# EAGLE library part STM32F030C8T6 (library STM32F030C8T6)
32-Bit MCU Cortex-M0 64KB Flash LQFP48 STM32F030C8T6, 32 bit ARM Cortex M0 Microcontroller 48MHz 64 kB Flash, 8 kB RAM, I2C 48-Pin LQFP Source: Datasheet
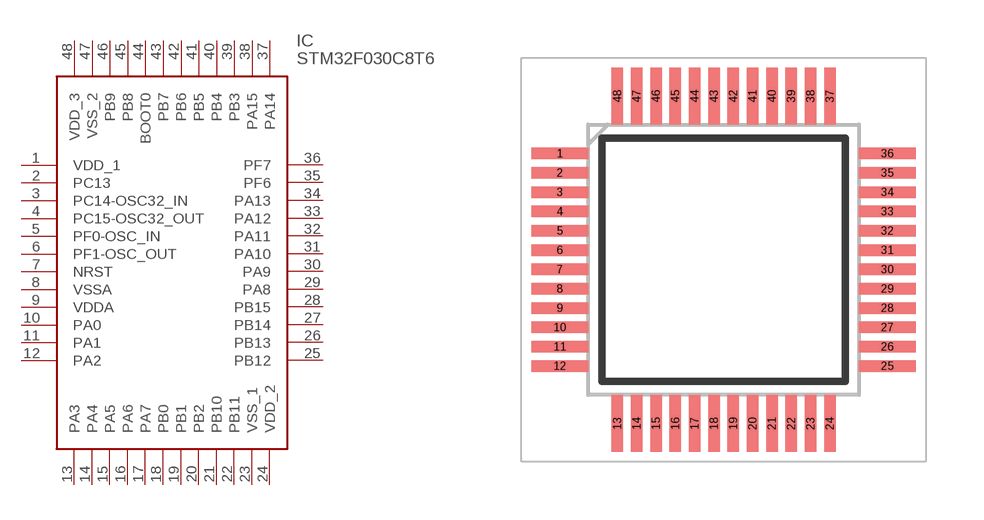
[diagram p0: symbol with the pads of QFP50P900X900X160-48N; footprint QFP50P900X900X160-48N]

Designator prefix IC

## STM32F030C8T6 (Arrow_Part_Number: STM32F030C8T6; Arrow_Price-Stock: https://www.arrow.com/en/products/stm32f030c8t6/stmicroelectronics; Description: 32-Bit MCU Cortex-M0 64KB Flash LQFP48 STM32F030C8T6, 32 bit ARM Cortex M0 Microcontroller 48MHz 64 kB Flash, 8 kB RAM, I2C 48-Pin LQFP; Height: 1.6mm; Manufacturer_Name: STMicroelectronics; Manufacturer_Part_Number: STM32F030C8T6; Mouser_Part_Number: 511-STM32F030C8T6; Mouser_Price-Stock: https://www.mouser.co.uk/ProductDetail/STMicroelectronics/STM32F030C8T6?qs=eyrSuY1LhL02NUjnPm0S4A%3D%3D)  [QFP50P900X900X160-48N]
1  VDD_1
2  PC13
3  PC14-OSC32_IN
4  PC15-OSC32_OUT
5  PF0-OSC_IN
6  PF1-OSC_OUT
7  NRST
8  VSSA
9  VDDA
10  PA0
11  PA1
12  PA2
13  PA3
14  PA4
15  PA5
16  PA6
17  PA7
18  PB0
19  PB1
20  PB2
21  PB10
22  PB11
23  VSS_1
24  VDD_2
25  PB12
26  PB13
27  PB14
28  PB15
29  PA8
30  PA9
31  PA10
32  PA11
33  PA12
34  PA13
35  PF6
36  PF7
37  PA14
38  PA15
39  PB3
40  PB4
41  PB5
42  PB6
43  PB7
44  BOOT0
45  PB8
46  PB9
47  VSS_2
48  VDD_3

## Footprint QFP50P900X900X160-48N (pad centres in mm)
LQFP48
smd 1.475 x 0.3: 1 -4.238,2.75; 2 -4.238,2.25; 3 -4.238,1.75; 4 -4.238,1.25; 5 -4.238,0.75; 6 -4.238,0.25; 7 -4.238,-0.25; 8 -4.238,-0.75; 9 -4.238,-1.25; 10 -4.238,-1.75; 11 -4.238,-2.25; 12 -4.238,-2.75; 25 4.238,-2.75; 26 4.238,-2.25; 27 4.238,-1.75; 28 4.238,-1.25; 29 4.238,-0.75; 30 4.238,-0.25; 31 4.238,0.25; 32 4.238,0.75; 33 4.238,1.25; 34 4.238,1.75; 35 4.238,2.25; 36 4.238,2.75
smd 0.3 x 1.475: 13 -2.75,-4.238; 14 -2.25,-4.238; 15 -1.75,-4.238; 16 -1.25,-4.238; 17 -0.75,-4.238; 18 -0.25,-4.238; 19 0.25,-4.238; 20 0.75,-4.238; 21 1.25,-4.238; 22 1.75,-4.238; 23 2.25,-4.238; 24 2.75,-4.238; 37 2.75,4.238; 38 2.25,4.238; 39 1.75,4.238; 40 1.25,4.238; 41 0.75,4.238; 42 0.25,4.238; 43 -0.25,4.238; 44 -0.75,4.238; 45 -1.25,4.238; 46 -1.75,4.238; 47 -2.25,4.238; 48 -2.75,4.238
